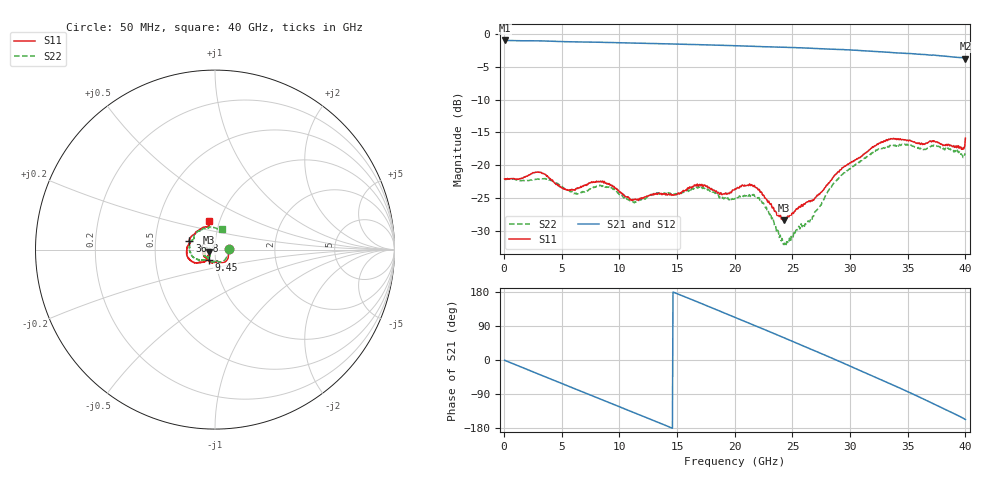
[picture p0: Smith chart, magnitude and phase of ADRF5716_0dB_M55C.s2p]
! Device: ADRF5716
! Description: 30GHz 2-Bit Digital Attenuator
! Frequency: 100 MHz – 30 GHz
! Ports:
! ATTIN  = Port 1
! ATTOUT = Port 2
! State: 0 dB Attenuation selected
! Supply Voltage:
! VDD  =  +3.30 Volts
! VSS  =  -3.30 Volts
! Control Voltages:
! D5 = 0V, D6 = 0V
! Temperature = -55 C
! Data: Data was collected using a calibrated network analyzer.
!  The reference plane is the package pins of ADRF5716 switch.
! Note: Analog Devices supplies this data as a sample of measured data for this product.
!  Your particular data for this product may vary.
!  Analog Devices reserves the right to change this data at anytime
# HZ S DB R 50
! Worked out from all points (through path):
!   800 points, 50 MHz to 40 GHz, reference 50 ohm
!   highest |S21| = -1.01 dB at 100 MHz (marker M1); lowest = -3.8 dB at 40 GHz (marker M2)
!   group delay of S21, straight-line fit = 35.4 ps
!   lowest |S11| = -28.3 dB at 24.25 GHz (marker M3), VSWR 1.08, Z = 46.5 - j1.31 ohm
!   |S11| at or under -10 dB: start of sweep to end of sweep
!   |S22| runs from -32.3 to -16.8 dB; largest |S21 - S12| = 0
!   S11 on the Smith chart (normalised r, x): 50 MHz: 1.17, +0.00; 9.45 GHz: 0.92, -0.11; 36.8 GHz: 0.75, +0.07; 40 GHz: 0.89, +0.29
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5e7  -22.08 1.2  -1.01 -0.6  -1.01 -0.6  -22.15 2.2
1e8  -22.04 -1.2  -1.01 -1.3  -1.01 -1.3  -22.12 -1.3
3.05e9  -21.01 -47.3  -1.07 -38.0  -1.07 -38.0  -22.13 -44.8
5.25e9  -23.54 -77.5  -1.19 -65.1  -1.19 -65.1  -23.61 -78.6
6.75e9  -23.25 -84.9  -1.24 -83.5  -1.24 -83.5  -24.13 -86.3
9.45e9  -23.24 -121.7  -1.33 -116.6  -1.33 -116.6  -23.66 -118.9
1.115e10  -25.21 -126.2  -1.41 -137.5  -1.41 -137.5  -25.55 -126.8
1.34e10  -24.27 -132.5  -1.49 -165.2  -1.49 -165.2  -24.19 -135.2
1.495e10  -24.40 -136.0  -1.56 175.7  -1.56 175.7  -24.46 -143.3
1.655e10  -23.04 -143.2  -1.63 156.0  -1.63 156.0  -23.48 -152.1
1.89e10  -24.46 -154.9  -1.75 126.6  -1.75 126.6  -24.98 -167.8
2.005e10  -23.54 -152.7  -1.81 112.1  -1.81 112.1  -25.02 -167.8
2.21e10  -23.65 -171.4  -1.93 86.3  -1.93 86.3  -24.90 174.5
2.425e10  -28.35 -158.4  -2.05 59.0  -2.05 59.0  -32.05 -174.2
2.67e10  -25.43 -135.8  -2.22 27.3  -2.22 27.3  -28.24 -131.6
2.835e10  -22.30 -128.0  -2.33 5.9  -2.33 5.9  -23.38 -129.7
2.99e10  -19.76 -136.2  -2.44 -14.7  -2.44 -14.7  -20.60 -141.4
3.335e10  -16.00 -164.2  -2.81 -61.1  -2.81 -61.1  -17.23 -175.0
3.515e10  -16.17 174.9  -3.00 -85.6  -3.00 -85.6  -16.83 162.5
3.68e10  -16.47 162.1  -3.22 -109.3  -3.22 -109.3  -17.31 149.6
3.845e10  -17.01 138.5  -3.42 -133.4  -3.42 -133.4  -17.44 123.3
4e10  -15.87 102.1  -3.78 -157.0  -3.78 -157.0  -18.20 70.4
